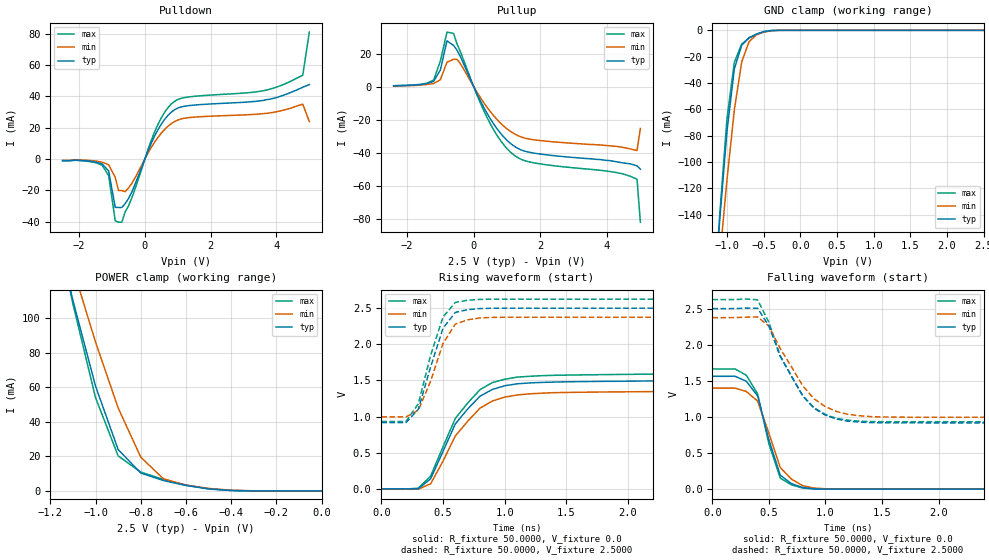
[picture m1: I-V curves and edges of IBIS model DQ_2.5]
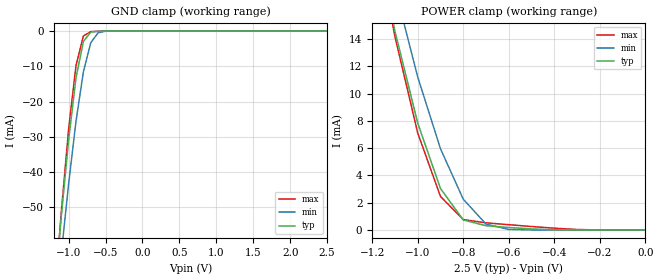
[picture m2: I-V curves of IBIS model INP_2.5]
|*** ISSI Synchronous Sram IBIS Model ***
[IBIS ver]	3.2
[File name]	is61vf204836b119bga.ibs
[File Rev]	1.0
[Date]	May 13,2013
[Notes]
|--- Version History --------------------------------
|1.0: prelimiary
[Disclaimer]	This information is for modeling purpose only
		and is not guaranteed
[Copyright]	INTEGRATED SILICON SOLUTION, INC. 2011
[Component]	IS61VF204836B_119BGA
[Manufacturer]	ISSI
[Package]
| variable   typ   min   max
R_pkg		100.34m			23.84m			218.59m
L_pkg		1.3400nH		0.3700nH		3.0300nH
C_pkg		41.410pF		0.4200pF		150.38pF
[Pin]  signal_name   model_name   R_pin   L_pin   C_pin
U7   VDDQ   POWER
U6   NC   NC
U5   TDO   DQ_2.5
U4   TCK   INP_2.5
U3   TDI   INP_2.5
U2   TMS   INP_2.5
U1   VDDQ   POWER
T7   ZZ   INP_2.5
T6   A   INP_2.5
T5   A   INP_2.5
T4   A   INP_2.5
T3   A   INP_2.5
T2   A   INP_2.5
T1   NC   NC
R7   NC   NC
R6   A   INP_2.5
R5   NC   NC
R4   VDD   POWER
R3   MODE   INP_2.5
R2   A   INP_2.5
R1   NC   NC
P7   DQa   DQ_2.5
P6   DQPa   DQ_2.5
P5   VSS   GND
P4   A0   INP_2.5
P3   VSS   GND
P2   DQPd   DQ_2.5
P1   DQd   DQ_2.5
N7   DQa   DQ_2.5
N6   DQa   DQ_2.5
N5   VSS   GND
N4   A1   INP_2.5
N3   VSS   GND
N2   DQd   DQ_2.5
N1   DQd   DQ_2.5
M7   VDDQ   POWER
M6   DQa   DQ_2.5
M5   VSS   GND
M4   BWEB   INP_2.5
M3   VSS   GND
M2   DQd   DQ_2.5
M1   VDDQ   POWER
L7   DQa   DQ_2.5
L6   DQa   DQ_2.5
L5   BWaB   INP_2.5
L4   NC   NC
L3   BWdB   INP_2.5
L2   DQd   DQ_2.5
L1   DQd   DQ_2.5
K7   DQa   DQ_2.5
K6   DQa   DQ_2.5
K5   VSS   GND
K4   CLK   INP_2.5
K3   VSS   GND
K2   DQd   DQ_2.5
K1   DQd   DQ_2.5
J7   VDDQ   POWER
J6   VDD   POWER
J5   NC   NC
J4   VDD   POWER
J3   NC   NC
J2   VDD   POWER
J1   VDDQ   POWER
H7   DQb   DQ_2.5
H6   DQb   DQ_2.5
H5   VSS   GND
H4   GWB   INP_2.5
H3   VSS   GND
H2   DQc   DQ_2.5
H1   DQc   DQ_2.5
G7   DQb   DQ_2.5
G6   DQb   DQ_2.5
G5   BWbB   INP_2.5
G4   ADVB   INP_2.5
G3   BWcB   INP_2.5
G2   DQc   DQ_2.5
G1   DQc   DQ_2.5
F7   VDDQ   POWER
F6   DQb   DQ_2.5
F5   VSS   GND
F4   OEB   INP_2.5
F3   VSS   GND
F2   DQc   DQ_2.5
F1   VDDQ   POWER
E7   DQb   DQ_2.5
E6   DQb   DQ_2.5
E5   VSS   GND
E4   CEB   INP_2.5
E3   VSS   GND
E2   DQc   DQ_2.5
E1   DQc   DQ_2.5
D7   DQb   DQ_2.5
D6   DQPb   DQ_2.5
D5   VSS   GND
D4   NC   NC
D3   VSS   GND
D2   DQPc   DQ_2.5
D1   DQc   DQ_2.5
C7   NC   Nc
C6   A   INP_2.5
C5   A   INP_2.5
C4   VDD   POWER
C3   A   INP_2.5
C2   A   INP_2.5
C1   NC   NC
B7   NC   NC
B6   A   INP_2.5
B5   A   INP_2.5
B4   ADSCB   INP_2.5
B3   A   INP_2.5
B2   A   INP_2.5
B1   NC   NC
A7   VDDQ   POWER
A6   A   INP_2.5
A5   A   INP_2.5
A4   ADSPB   INP_2.5
A3   A   INP_2.5
A2   A   INP_2.5
A1   VDDQ   POWER
| Models and submodels in the file (2): DQ_2.5 (3-state), INP_2.5 (Input)
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|   Model DQ_2.5
[Model]		DQ_2.5
Model_type	3-state
Polarity   Non-Inverting
Enable   Active-Low
Vmeas = 	0.7500V
Cref = 		5.0000pF
Rref = 		50.0000
Vref = 		1.2500V
C_comp   3.8290pF   3.3420pF   4.0300pF|
[Temperature Range]	  25.0000   100.0000   0.0
[Voltage Range]   2.5000V   2.3750V   2.6250V
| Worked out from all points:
|   slope of the pulldown table from 0 to 0.375 V, typ, clamps not added: 21.1 ohm
|   slope of the pullup table from 0 to 0.375 V, typ, clamps not added: 24.7 ohm
|   GND clamp passes 1 mA (typ) near -0.49 V on its own axis
|   POWER clamp passes 1 mA (typ) near -0.48 V on its own axis
|   rising waveform, R_fixture 50.0000, V_fixture 0.0: 20-80 % time 314ps typ, 320ps min, 316ps max; typ from 0 V to 1.51 V
|   rising waveform, R_fixture 50.0000, V_fixture 2.5000: 20-80 % time 170ps typ, 187ps min, 169ps max; typ from 0.918 V to 2.5 V
|   falling waveform, R_fixture 50.0000, V_fixture 0.0: 20-80 % time 169ps typ, 190ps min, 167ps max; typ from 1.56 V to 0 V
|   falling waveform, R_fixture 50.0000, V_fixture 2.5000: 20-80 % time 314ps typ, 336ps min, 308ps max; typ from 2.5 V to 0.918 V
[Pulldown]
|Voltage	  I(typ)   I(min)   I(max)
-2.5V     -1mA       -900uA     -1.1mA
-1.3V     -3.1mA     -1.98mA    -3.85mA
-1.1V     -7.6mA     -3.69mA    -10.56mA
-900mV    -30.82mA   -11.68mA   -39.46mA
-800mV    -30.93mA   -20.13mA   -40.31mA
-700mV    -30.93mA   -20.13mA   -40.31mA
-400mV    -21.21mA   -15.69mA   -25.04mA
300mV     14.77mA    10.9mA     17.5mA
800mV     29.84mA    22.52mA    35.05mA
3.7V      37.9mA     29.16mA    43.99mA
4.8V      45.8mA     35.01mA    53.46mA
5V        47.5mA     23.97mA    81.01mA
[Pullup]
|Voltage	  I(typ)   I(min)   I(max)
-2.4V     400uA      360uA      550uA
-1.2V     3.2mA      1.89mA     3.96mA
-1V       9.97mA     4.104mA    15.48mA
-800mV    27.74mA    14.77mA    33.01mA
-600mV    24.84mA    16.54mA    32.14mA
-400mV    18.24mA    13.88mA    21.25mA
300mV     -12.46mA   -9.666mA   -14.47mA
1V        -32.57mA   -25.6mA    -37.58mA
1.6V      -39.48mA   -31.55mA   -45.26mA
4.1V      -44.9mA    -35.91mA   -51.48mA
4.9V      -48mA      -38.7mA    -56.1mA
5V        -50mA      -25.39mA   -82.14mA
[GND_clamp]
|Voltage	  I(typ)   I(min)   I(max)
-2.5V     -1.238A    -1.081A    -1.377A
-1.2V     -220.2mA   -237.3mA   -225.5mA
-1.1V     -144.4mA   -173.5mA   -140.5mA
-1V       -76.37mA   -113.2mA   -66.76mA
-900mV    -29.2mA    -60.35mA   -24.24mA
-800mV    -11.34mA   -23.99mA   -10.52mA
-700mV    -5.573mA   -8.7mA     -5.892mA
-600mV    -2.907mA   -3.457mA   -3.011mA
-500mV    -1.075mA   -1.408mA   -999.8uA
-300mV    -9.492uA   -41.34uA   -5.052uA
2.5V      40.97nA    416.1nA    43nA
[POWER_clamp]
|Voltage	  I(typ)   I(min)   I(max)
-2.5V     946.2mA    803.1mA    1.061A
-1.2V     165.2mA    174.2mA    170.3mA
-1.1V     110.4mA    129mA      108.4mA
-1V       60.76mA    86.26mA    54.07mA
-900mV    23.99mA    48.12mA    20.31mA
-800mV    10.36mA    19.57mA    10.92mA
-700mV    6.025mA    7.051mA    6.647mA
-600mV    3.142mA    3.321mA    3.423mA
-500mV    1.147mA    1.448mA    1.242mA
-400mV    194.4uA    400.6uA    266.4uA
0V        40.97nA    40.9nA     75.05nA
[Ramp]
| variable   typ   min   max
dV/dt_r		0.9042/0.2795n   0.7824/0.2922n   0.9954/0.2697n
dV/dt_f		0.9493/0.2827n   0.8275/0.2702n   1.0156/0.3061n
R_load =	50.0000
[Rising Waveform]
R_fixture=	50.0000
V_fixture=	0.0
V_fixture_min=	0.0
V_fixture_max=	0.0
|time   V(typ)   V(min)   V(max)
0s        0V         0V         0V
300ps     3.703mV    -2.782mV   10.28mV
400ps     140.9mV    71.68mV    179.8mV
600ps     899.4mV    732.5mV    975.4mV
800ps     1.282V     1.117V     1.373V
900ps     1.375V     1.216V     1.47V
1ns       1.427V     1.27V      1.516V
1.2ns     1.466V     1.315V     1.557V
1.6ns     1.484V     1.337V     1.577V
5ns       1.507V     1.359V     1.602V
[Rising Waveform]
R_fixture=	50.0000
V_fixture=	2.5000
V_fixture_min=	2.3750
V_fixture_max=	2.6250
|time   V(typ)   V(min)   V(max)
0s        917.8mV    995.8mV    932.4mV
200ps     917.8mV    995.8mV    932.6mV
300ps     1.101V     1.087V     1.177V
400ps     1.689V     1.492V     1.849V
500ps     2.221V     2.011V     2.377V
600ps     2.441V     2.279V     2.579V
700ps     2.478V     2.338V     2.608V
800ps     2.494V     2.365V     2.621V
900ps     2.498V     2.372V     2.623V
5ns       2.5V       2.375V     2.625V
[Falling Waveform]
R_fixture=	50.0000
V_fixture=	0.0
V_fixture_min=	0.0
V_fixture_max=	0.0
|time   V(typ)   V(min)   V(max)
0s        1.563V     1.4V       1.665V
200ps     1.563V     1.399V     1.665V
300ps     1.495V     1.353V     1.577V
400ps     1.292V     1.22V      1.321V
500ps     684mV      773.4mV    627.2mV
600ps     194.2mV    300.3mV    154.3mV
700ps     76.23mV    138.2mV    59.74mV
800ps     22.14mV    46.86mV    14.45mV
1.1ns     594.5uV    1.764mV    405.6uV
5ns       23.76uV    34.03uV    20.31uV
[Falling Waveform]
R_fixture=	50.0000
V_fixture=	2.5000
V_fixture_min=	2.3750
V_fixture_max=	2.6250
|time   V(typ)   V(min)   V(max)
0s        2.5V       2.375V     2.625V
400ps     2.505V     2.385V     2.622V
500ps     2.259V     2.258V     2.31V
600ps     1.839V     1.948V     1.847V
800ps     1.289V     1.429V     1.292V
900ps     1.119V     1.25V      1.126V
1ns       1.024V     1.142V     1.033V
1.1ns     969.7mV    1.075V     979.6mV
1.5ns     919.4mV    999.8mV    933.8mV
5ns       917.8mV    995.8mV    932.4mV
|   Model INP_2.5
[Model]		INP_2.5
Model_type	Input
Polarity   Non-Inverting
Enable   Active-Low
Vinl = 		0.8000V
Vinh = 		2.0000V
C_comp   3.8290pF   3.3420pF   4.0300pF|
[Temperature Range]	  25.0000   100.0000   0.0
[Voltage Range]   2.5000V   2.3750V   2.6250V
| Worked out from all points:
|   GND clamp passes 1 mA (typ) near -0.73 V on its own axis
|   POWER clamp passes 1 mA (typ) near -0.81 V on its own axis
[GND_clamp]
|Voltage	  I(typ)   I(min)   I(max)
-2.5V     -434.7mA   -399mA     -475.2mA
-1.2V     -76.89mA   -84.89mA   -78.19mA
-1.1V     -52.83mA   -63.46mA   -51.66mA
-1V       -30.98mA   -43.42mA   -27.92mA
-900mV    -13.28mA   -25.61mA   -9.811mA
-800mV    -2.971mA   -11.61mA   -1.401mA
-700mV    -287uA     -3.303mA   -148.3uA
-600mV    -52.18uA   -480.7uA   -48.72uA
-500mV    -11.21uA   -45.78uA   -9.079uA
2.5V      40.19nA    40.4nA     42.61nA
[POWER_clamp]
|Voltage	  I(typ)   I(min)   I(max)
-2.5V     189.7mA    171.9mA    207.8mA
-1.2V     22.77mA    25.28mA    23.03mA
-1.1V     14.57mA    17.73mA    14.18mA
-1V       7.84mA     11.21mA    7.108mA
-900mV    3.038mA    5.954mA    2.453mA
-800mV    736uA      2.255mA    762.7uA
-700mV    308.2uA    432.8uA    524.6uA
-600mV    181.1uA    36.29uA    386.3uA
-400mV    10.09uA    187.6nA    130.9uA
-300mV    415nA      89.24nA    33.9uA
0V        40.19nA    23.22nA    74.57nA
